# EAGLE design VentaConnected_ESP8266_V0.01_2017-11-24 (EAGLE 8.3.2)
VERSION: 0.01
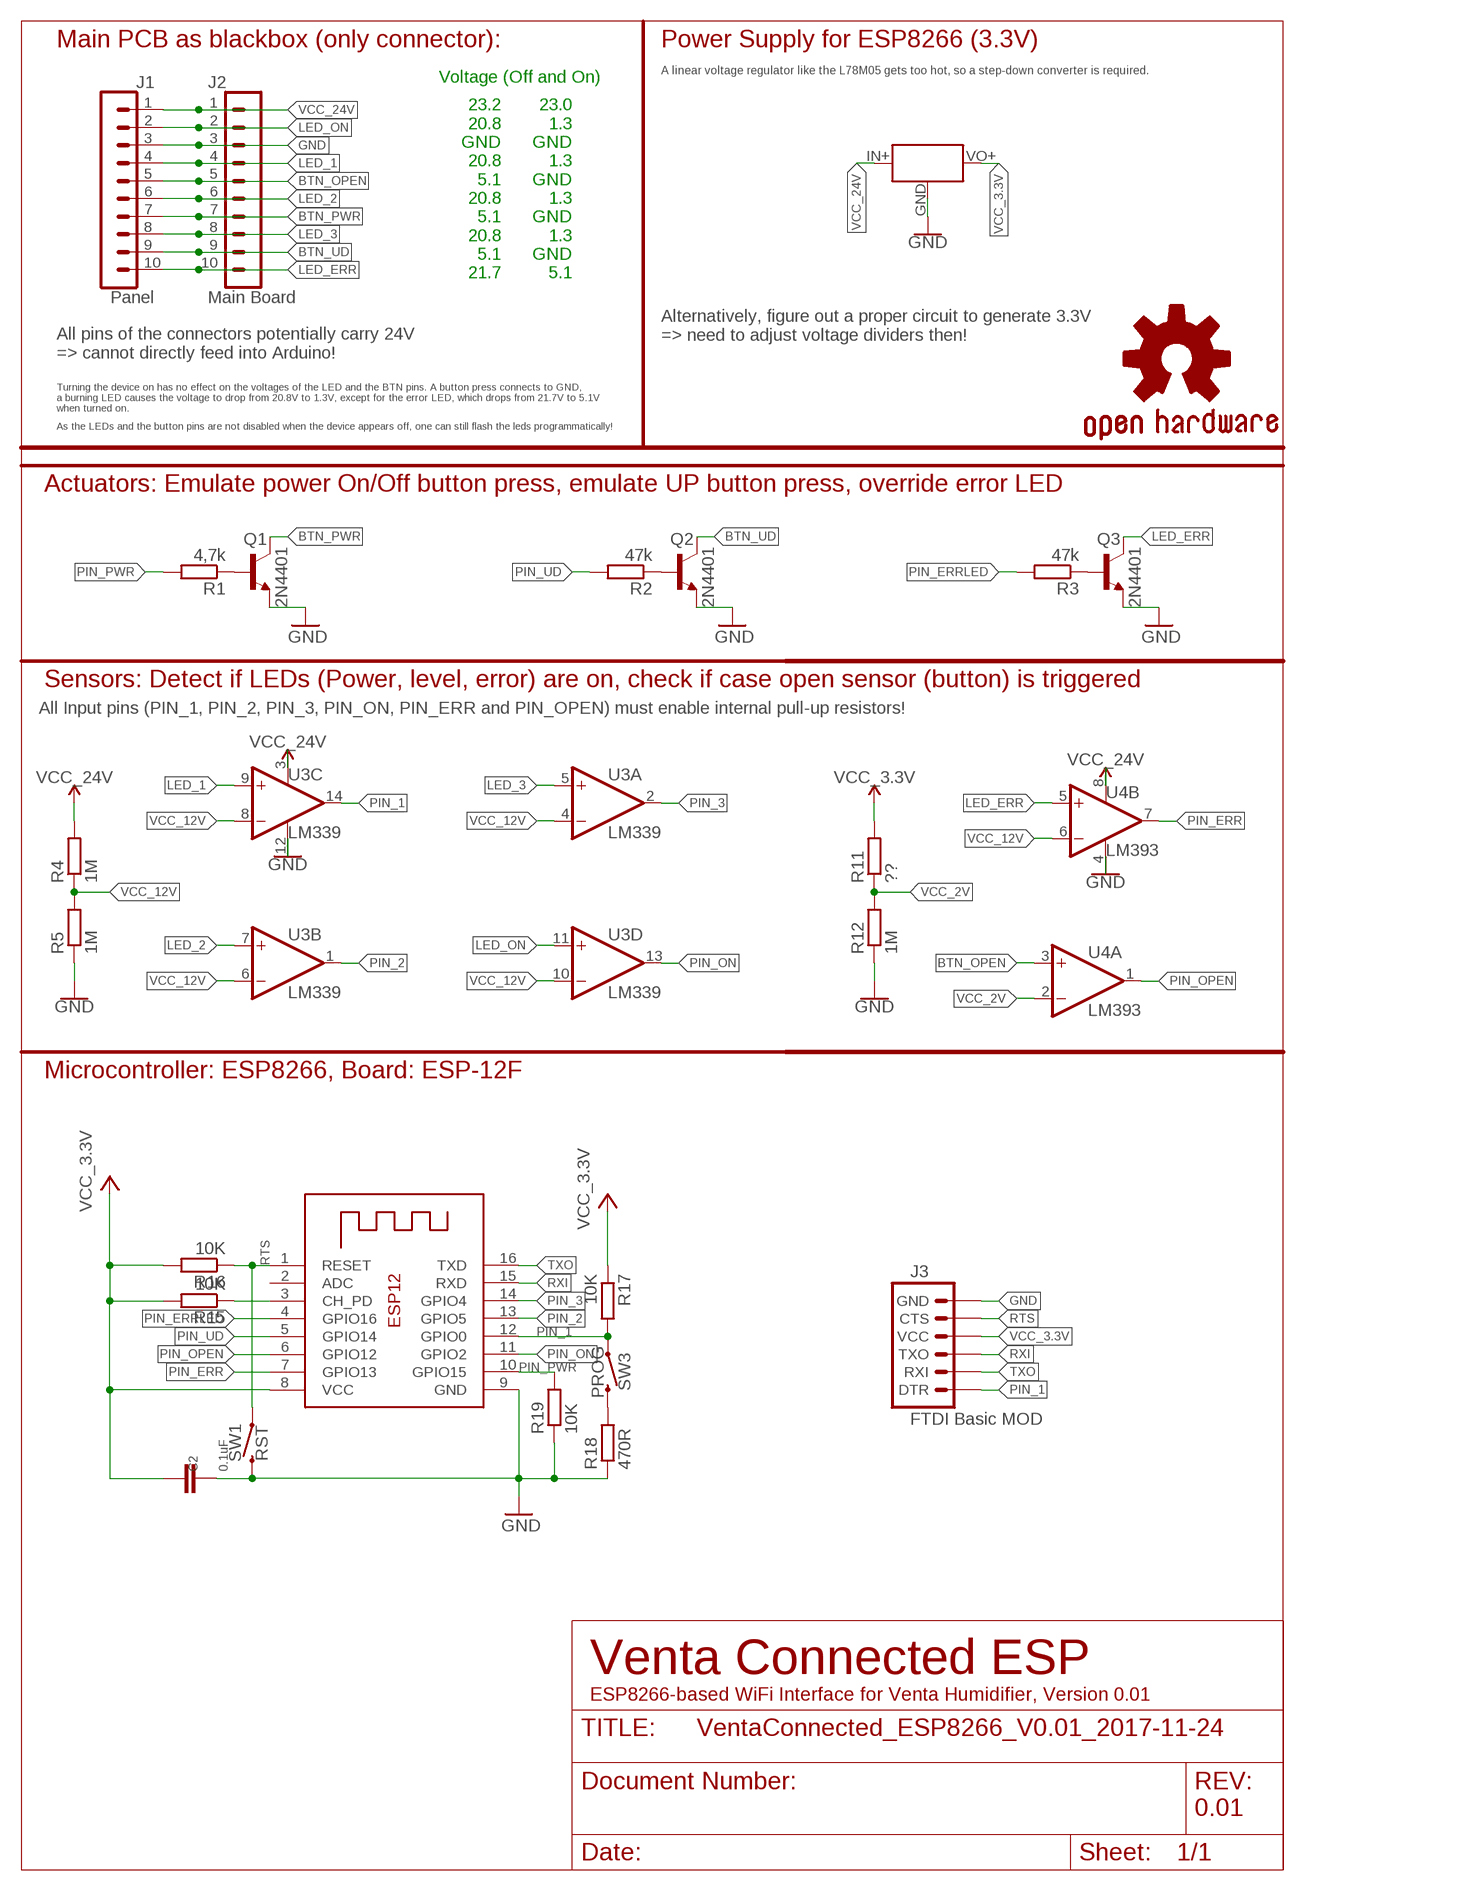
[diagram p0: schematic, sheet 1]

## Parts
C2  0.1uF  C-EUC0805  [C0805]
GOLD_ORB_SM1  OSHWLOGO_GOLD_ORB_SM  [OSHW2]
J1  Panel  CONN_05X2SHD  [2X5-SHROUDED]
J2  Main Board  CONN_05X2PTH  [2X5]
J3  FTDI Basic MOD  ARDUINO_SERIAL_PROGRAMPTH  [1X06]
Q1  2N4401  MMBT4401LT1-NPN-SOT23-BEC  [SOT23-BEC]
Q2  2N4401  MMBT4401LT1-NPN-SOT23-BEC  [SOT23-BEC]
Q3  2N4401  MMBT4401LT1-NPN-SOT23-BEC  [SOT23-BEC]
R1  4,7k  R-EU_R0805  [R0805]
R2  47k  R-EU_R0805  [R0805]
R3  47k  R-EU_R0805  [R0805]
R4  1M  R-EU_R0805  [R0805]
R5  1M  R-EU_R0805  [R0805]
R11  ??  R-EU_R0805  [R0805]
R12  1M  R-EU_R0805  [R0805]
R15  10K  R-EU_R0805  [R0805]
R16  10K  R-EU_R0805  [R0805]
R17  10K  R-EU_R0805  [R0805]
R18  470R  R-EU_R0805  [R0805]
R19  10K  R-EU_R0805  [R0805]
SW1  RST  MOMENTARY-SWITCH-SPST-SMD-6.0X3.5MM  [TACTILE_SWITCH_SMD_6.0X3.5MM]
SW3  PROG  MOMENTARY-SWITCH-SPST-SMD-6.0X3.5MM  [TACTILE_SWITCH_SMD_6.0X3.5MM]
U2  3.3V_BUCK_CONVERTER  MINI_BUCK_CONVERTER_UPSIDEDOWN  [MINI_BUCK_CONVERTER_UPDOWN]
U3  LM339  TLC339D  [SO14]
U4  LM393  LM393D  [SO08]
X2  ESP-12e  ESP-12  [ESP-12]

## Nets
BTN_OPEN: J1.5 J2.5 U4.3(A:+IN)
BTN_PWR: J1.7 J2.7 Q1.C
BTN_UD: J1.9 J2.9 Q2.C
CH_PD: R15.1 X2.3(CH_PD)
GND: C2.1 J1.3 J2.3 J3.6(GND) Q1.E Q2.E Q3.E R5.1 R12.1 R18.1 R19.1 SW1.2 U2.GND U3.12(P:V-) U4.4(P:V-) X2.9(GND)
LED_1: J1.4 J2.4 U3.9(C:+IN)
LED_2: J1.6 J2.6 U3.7(B:+IN)
LED_3: J1.8 J2.8 U3.5(A:+IN)
LED_ERR: J1.10 J2.10 Q3.C U4.5(B:+IN)
LED_ON: J1.2 J2.2 U3.11(D:+IN)
N$2: Q1.B R1.1
N$4: R18.2 SW3.2
N$5: Q3.B R3.1
N$6: Q2.B R2.1
PIN_1: J3.1(DTR) R17.2 SW3.1 U3.14(C:OUT) X2.12(GPIO0)
PIN_2: U3.1(B:OUT) X2.13(GPIO5)
PIN_3: U3.2(A:OUT) X2.14(GPIO4)
PIN_ERR: U4.7(B:OUT) X2.7(GPIO13)
PIN_ERRLED: R3.2 X2.4(GPIO16)
PIN_ON: U3.13(D:OUT) X2.11(GPIO2)
PIN_OPEN: U4.1(A:OUT) X2.6(GPIO12)
PIN_PWR: R1.2 R19.2 X2.10(GPIO15)
PIN_UD: R2.2 X2.5(GPIO14)
RTS: J3.5(CTS) R16.1 SW1.1 X2.1(RESET)
RXI: J3.3(TXO) X2.15(RXD)
TXO: J3.2(RXI) X2.16(TXD)
VCC_2V: R11.1 R12.2 U4.2(A:-IN)
VCC_3.3V: C2.2 J3.4(VCC) R11.2 R15.2 R16.2 R17.1 U2.VO+(VOUT) X2.8(VCC)
VCC_12V: R4.1 R5.2 U3.4(A:-IN) U3.6(B:-IN) U3.8(C:-IN) U3.10(D:-IN) U4.6(B:-IN)
VCC_24V: J1.1 J2.1 R4.2 U2.IN+(VIN) U3.3(P:V+) U4.8(P:V+)
Unconnected: X2.2(ADC)

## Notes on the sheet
- Main PCB as blackbox (only connector): | Power Supply for ESP8266 (3.3V)
- A linear voltage regulator like the L78M05 gets too hot, so a step-down converter is required.
- Voltage (Off and On)
- 23.2
  20.8
  GND
  20.8
  5.1
  20.8
  5.1
  20.8
  5.1
  21.7
- 23.0
  1.3
  GND
  1.3
  GND
  1.3
  GND
  1.3
  GND
  5.1
- Alternatively, figure out a proper circuit to generate 3.3V 
  => need to adjust voltage dividers then!
- All pins of the connectors potentially carry 24V 
  => cannot directly feed into Arduino!
- Turning the device on has no effect on the voltages of the LED and the BTN pins. A button press connects to GND, 
  a burning LED causes the voltage to drop from 20.8V to 1.3V, except for the error LED, which drops from 21.7V to 5.1V 
  when turned on.
- As the LEDs and the button pins are not disabled when the device appears off, one can still flash the leds programmatically!
- Actuators: Emulate power On/Off button press, emulate UP button press, override error LED
- Sensors: Detect if LEDs (Power, level, error) are on, check if case open sensor (button) is triggered
- All Input pins (PIN_1, PIN_2, PIN_3, PIN_ON, PIN_ERR and PIN_OPEN) must enable internal pull-up resistors!
- Microcontroller: ESP8266, Board: ESP-12F
- Venta Connected ESP
- ESP8266-based WiFi Interface for Venta Humidifier, Version 0.01

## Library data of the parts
C2 = resistor:C-EU: CAPACITOR, European symbol
GOLD_ORB_SM1 = bfl:OSHWLOGO: These are Open-Source Hardware logos.
J1 = opentools-connectors:CONN_05X2: Multi connection point. Often used as Generic Header-pin footprint for 0.1 inch spaced/style header connections For AVR SPI programming port, see special device with nice symbol: "AVR_SPI_PROG_5x2.dev" You can populate with any combo of single row headers, but if you'd like an exact match, check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; PROD_ID: CONN-08671; SF_ID: PRT-08506
J2 = opentools-connectors:CONN_05X2: Multi connection point. Often used as Generic Header-pin footprint for 0.1 inch spaced/style header connections For AVR SPI programming port, see special device with nice symbol: "AVR_SPI_PROG_5x2.dev" You can populate with any combo of single row headers, but if you'd like an exact match, check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; PROD_ID: CONN-08499; SF_ID: PRT-0778
J3 = SparkFun:ARDUINO_SERIAL_PROGRAM
Q1-Q3 = transistor-neu-to92:*-NPN-: NPN Transistror
R1-R5 R11 R12 = resistor:R-EU_: RESISTOR, European symbol
R15-R19 = rcl:R-EU_: RESISTOR, European symbol
SW1 SW3 = SparkFun-Switches:MOMENTARY-SWITCH-SPST: Momentary Switch (Pushbutton) - SPST; PROD_ID: SWCH-00815; SF_SKU: COM-08229
U2 = opentools-sensors:MINI_BUCK_CONVERTER: 4.5-40V Step Down Buck Converter
U3 = linear:TLC339: COMPARATOR
U4 = linear:LM393: COMPARATOR
X2 = adafruit:ESP-12

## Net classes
0 default: width 0.203 mm
1 vcc: width 0.254 mm

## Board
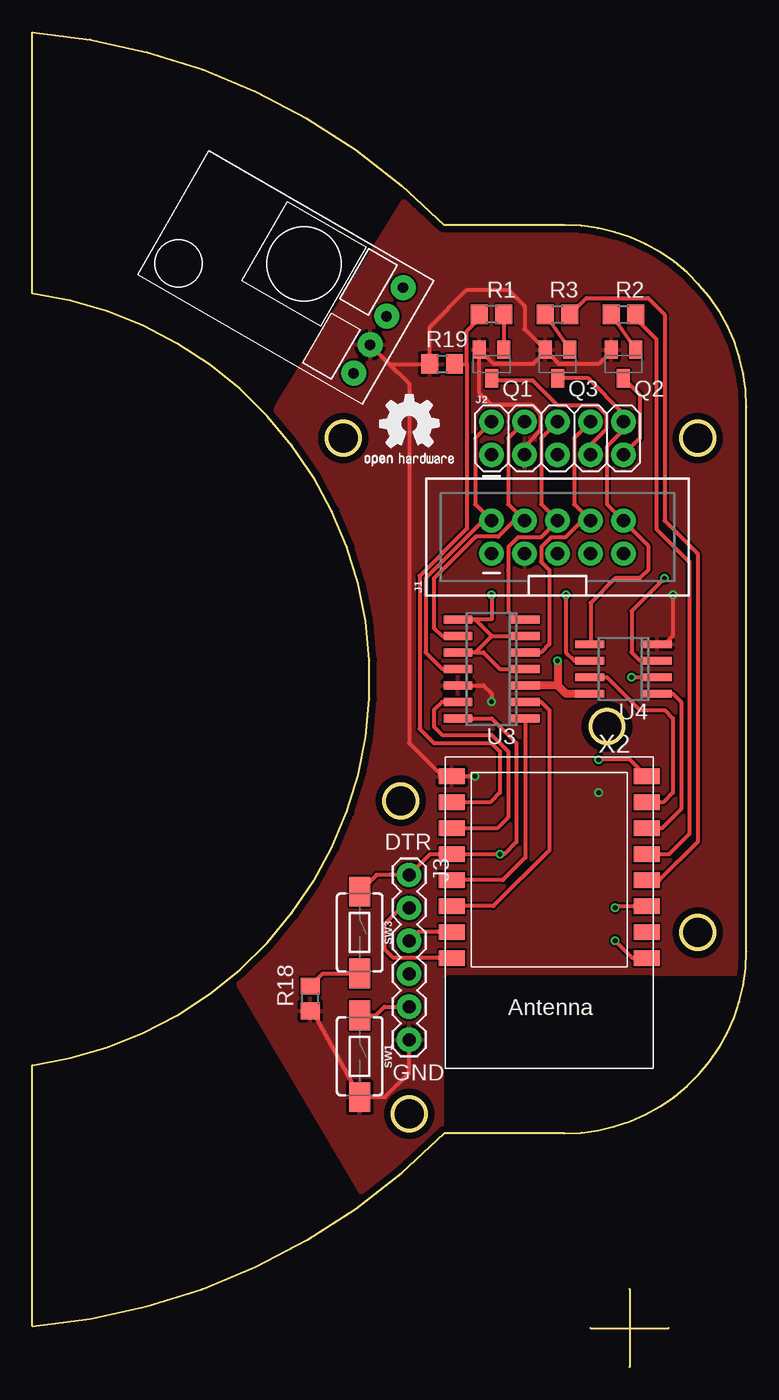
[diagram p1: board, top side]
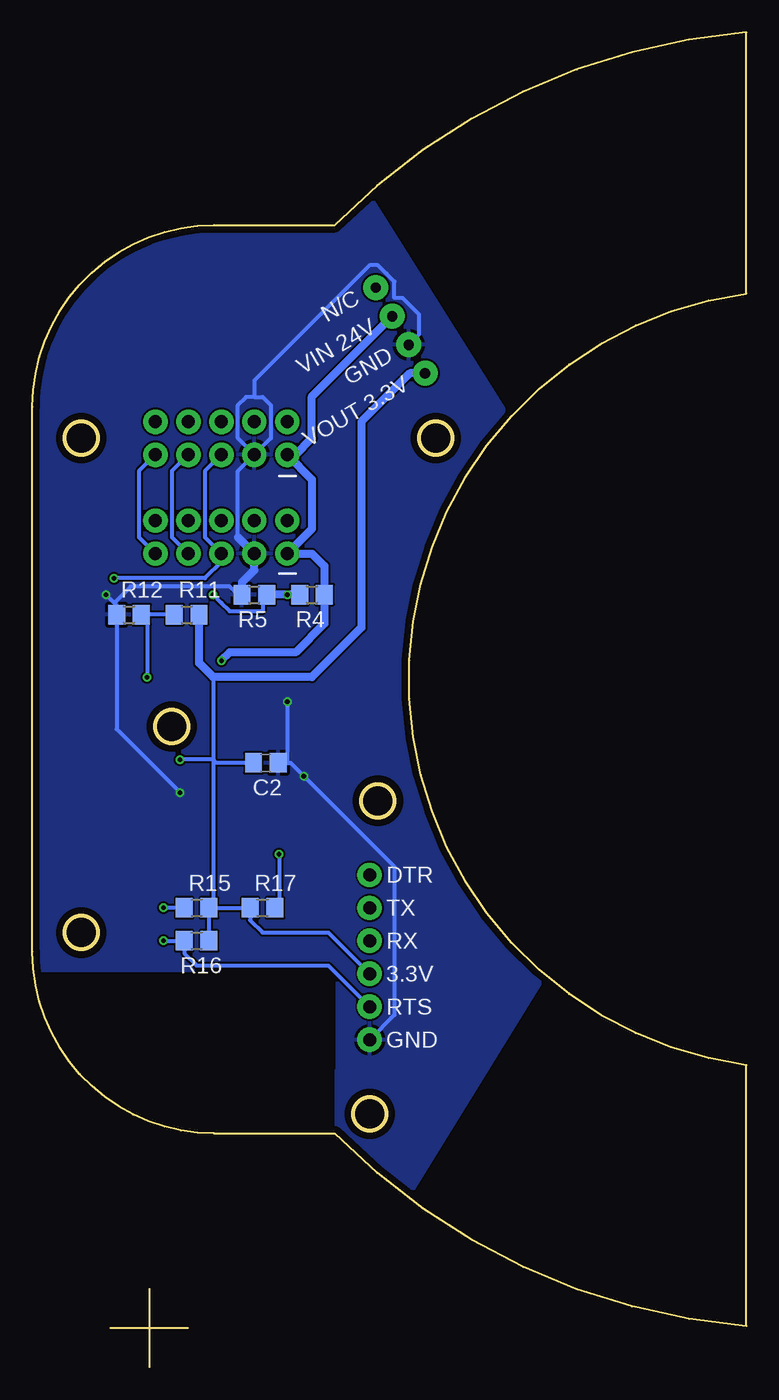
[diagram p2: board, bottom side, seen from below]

Size 55 x 102.85 mm. Coordinates in mm from the lower left corner, seen from the top.
Outline: 46,6 46,0
Outline: 43,3 49,3
Outline: 41,18 arc90 55,32 55,74 arc90 41,88 31.71,88 arc41 0,102.85 0,82.73 arc-165 0,23.27 0,3.16 arc41 31.71,18 41,18
Outline: circle at 29.02,19.51 radius 1.27
Outline: circle at 51.24,33.48 radius 1.27
Outline: circle at 28.38,43.64 radius 1.27
Outline: circle at 51.24,71.58 radius 1.27
Outline: circle at 23.94,71.58 radius 1.27
Outline: circle at 44.26,49.35 radius 1.27
Copper layers (1*16): Top 0.035mm / dielectric 1.6mm / Bottom 0.035mm
Design rules "Elecrow_2-layer_PCB_eagle_rule": minimum track width 6mil, minimum drill 12mil, track to track 6mil, track to pad 6mil, pad to pad 6mil, via to via 8mil, smd to smd 0mil, copper to edge 20mil, drill to drill 10mil, minimum pad ring 6mil, minimum via ring 6mil, stop-mask expansion 0mil, vias tented up to drill 100mil, thermal gap 10mil

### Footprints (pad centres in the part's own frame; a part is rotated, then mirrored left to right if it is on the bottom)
C0805 = smd 1.3 x 1.5: 1 -0.95,0; 2 0.95,0
2X5-SHROUDED = drill 1.016 pad 1.88: 1 -1.27,5.08; 2 1.27,5.08; 3 -1.27,2.54; 4 1.27,2.54; 5 -1.27,0; 6 1.27,0; 7 -1.27,-2.54; 8 1.27,-2.54; 9 -1.27,-5.08; 10 1.27,-5.08
2X5 = drill 1.016 pad 1.88: 1 0,0; 2 0,2.54; 3 2.54,0; 4 2.54,2.54; 5 5.08,0; 6 5.08,2.54; 7 7.62,0; 8 7.62,2.54; 9 10.16,0; 10 10.16,2.54
1X06 = drill 1.016 pad 1.88: 1 0,0; 2 2.54,0; 3 5.08,0; 4 7.62,0; 5 10.16,0; 6 12.7,0
SOT23-BEC = smd 1 x 1.4: B -0.95,-1.1; C 0,1.1; E 0.95,-1.1
R0805 = smd 1.3 x 1.5: 1 -0.95,0; 2 0.95,0
TACTILE_SWITCH_SMD_6.0X3.5MM = smd 2.3 x 1.6: 1 -3.15,0; 2 3.15,0
MINI_BUCK_CONVERTER_UPDOWN = drill 0.8 pad 1.93: EN -1.27,1.27; GND -6.35,1.27; IN+ -3.81,1.27; VO+ -8.89,1.27
SO14 = smd 0.6 x 2.2: 1 -3.81,-2.6; 2 -2.54,-2.6; 3 -1.27,-2.6; 4 0,-2.6; 5 1.27,-2.6; 6 2.54,-2.6; 7 3.81,-2.6; 8 3.81,2.6; 9 2.54,2.6; 10 1.27,2.6; 11 0,2.6; 12 -1.27,2.6; 13 -2.54,2.6; 14 -3.81,2.6
SO08 = smd 0.6 x 2.2: 1 -1.905,-2.6; 2 -0.635,-2.6; 3 0.635,-2.6; 4 1.905,-2.6; 5 1.905,2.6; 6 0.635,2.6; 7 -0.635,2.6; 8 -1.905,2.6
ESP-12 = smd 2 x 1.2: 1 -7.5,4.5; 2 -7.5,2.5; 3 -7.5,0.5; 4 -7.5,-1.5; 5 -7.5,-3.5; 6 -7.5,-5.5; 7 -7.5,-7.5; 8 -7.5,-9.5; 9 7.5,-9.5; 10 7.5,-7.5; 11 7.5,-5.5; 12 7.5,-3.5; 13 7.5,-1.5; 14 7.5,0.5; 15 7.5,2.5; 16 7.5,4.5

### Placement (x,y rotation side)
C2  37.02,46.56 180 bottom
GOLD_ORB_SM1  25.21,68.41 0 top
J1  40.45,63.96 90 top
J2  35.37,70.31 0 top
J3  29.02,37.92 270 top
Q1  35.37,77.3 180 top
Q2  45.53,77.3 180 top
Q3  40.45,77.3 180 top
R1  35.37,81.11 180 top
R2  45.53,81.11 0 top
R3  40.45,81.11 0 top
R4  33.47,59.52 0 bottom
R5  37.91,59.52 0 bottom
R11  43.12,57.99 0 bottom
R12  47.56,57.99 0 bottom
R15  42.35,35.38 0 bottom
R16  42.35,32.84 0 bottom
R17  37.27,35.38 0 bottom
R18  21.4,28.4 90 top
R19  31.56,77.3 0 top
SW1  25.21,23.95 270 top
SW3  25.21,33.48 270 top
U2  30.29,83.64 60 top
U3  35.37,53.8 90 top
U4  45.53,53.8 90 top
X2  39.81,36.02 180 top

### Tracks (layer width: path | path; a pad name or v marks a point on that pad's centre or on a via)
BTN_OPEN  (via drill 0.35)
  Top 0.305: v48.7,60.78 46.16,58.24 46.16,55.07 46.8,54.44 U4.3
  Bottom 0.305: J2.5 41.72,69.04 41.72,63.96 J1.5 40.45,62.05 41.72,60.78 v48.7,60.78
BTN_PWR
  Top 0.305: Q1.C 35.54,76.03 38.55,76.03 40.48,74.09 43.51,74.09 44.23,73.37 44.23,72.33 42.99,71.09 J2.7
  Bottom 0.305: J2.7 44.26,69.04 44.26,63.96 J1.7
BTN_UD
  Top 0.305: 45.53,76.03 Q2.C 46.8,74.92 46.8,71.58 J2.9
  Bottom 0.305: J2.9 46.8,69.04 46.8,63.96 J1.9
CH_PD  (via drill 0.35)
  Top 0.305: v44.9,35.38 45.03,35.52 X2.3
  Bottom 0.305: R15.1 v44.9,35.38
GND  (via drill 0.35)
  Top 0.305: 32.34,45.55 v34.1,45.55 | 32.34,45.55 X2.9 | R18.1 21.75,27.11 SW1.2 27.14,20.8 29.02,22.68 J3.6 | J2.3 37.91,70.94 38.72,71.76 38.72,71.77 39.17,72.22 39.17,73.49 38.55,74.12 35.37,74.12 34.42,75.07 Q1.E 35.52,77.3 38.55,77.3 39.5,78.25 Q3.E 39.57,78.32 | v49.34,59.52 49.34,56.34 48.7,55.7 U4.4 | U3.12 34.73,52.53 35.37,51.9 v35.37,51.26 | Q2.E 44.58,78.25 43.62,77.3 40.6,77.3 39.57,78.32 | U2.GND 27.31,77.49 | 27.31,77.49 27.5,77.3 R19.1 30.61,80.16 33.47,83.01 36.64,83.01 37.91,81.74 37.91,79.98 39.57,78.32 | 27.31,77.49 29.02,75.78 29.02,48.09 31.56,45.55 32.34,45.55
  Bottom 0.305: J2.3 39.18,69.04 39.18,63.96 | 35.37,46.56 C2.1 | 35.37,46.56 35.12,46.56 v34.1,45.55 27.11,38.56 27.11,27.13 J3.6 | J2.3 39.18,71.58 39.18,74.12 38.55,74.75 37.91,74.75 | J2.3 36.64,71.58 36.64,74.12 37.27,74.75 37.91,74.75 | v35.37,51.26 35.37,46.56 | 48.7,58.88 48.51,58.69 R12.1 48.51,49.16 v43.62,44.27 | 48.7,58.88 v49.34,59.52 | R5.1 39.18,59.52 39.81,60.15 47.44,60.15 48.7,58.88 | U2.GND 25.21,79.59 25.21,81.11 26.48,82.38 27.11,82.38 27.11,83.64 27.69,84.22 27.72,84.27 27.75,84.28 28.38,84.92 29.02,84.92 37.91,76.03 37.91,74.75
  Bottom 0.61: R5.1 38.86,60.47 37.91,61.42 J1.3 39.18,63.96
  pour Top (isolate 0.152): 29.02,90.63 18.86,74.12 18.23,72.85 22.04,67.14 24.57,62.05 25.84,53.8 25.21,46.18 20.77,36.02 15.68,29.67 25.84,12.53 31.56,16.97 31.56,30.3 55.05,30.3 55.69,74.12 51.88,84.28 42.99,88.09 31.56,88.09
  pour Bottom (isolate 0.152): 29.02,90.25 18.23,73.1 20.13,69.93 23.94,62.31 25.84,55.32 25.21,45.8 19.5,34.37 15.68,29.92 25.84,13.41 29.02,15.32 31.56,17.86 31.56,30.56 55.05,30.56 55.69,73.74 51.88,83.9 42.99,87.71 31.56,87.71
LED_1
  Top 0.305: J2.4 36.64,71.58 36.64,66.5 J1.4 37.13,65.23 35.89,63.98 34.14,63.98 34.11,63.95 | 34.11,63.95 34.11,63.96 | 34.11,63.95 30.93,60.78 30.93,56.97 31.56,56.34 U3.9
LED_2
  Top 0.305: J2.6 39.18,71.58 39.18,66.5 J1.6 39.16,63.94 37.39,63.94 36.66,63.21 36.66,61.45 | 36.64,61.42 36.66,61.45 | 36.66,61.45 36.66,58.22 37.27,57.61 U3.7
LED_3
  Top 0.305: J2.8 41.72,71.58 41.72,66.5 J1.8 42.35,65.23 41.06,63.94 39.93,63.94 39.2,63.21 39.2,62.08 39.18,62.05 39.81,61.42 39.81,55.7 39.18,55.07 U3.5
LED_ERR
  Top 0.305: Q3.C 42.82,76.19 45.53,73.48 J2.10 45.53,72.22 44.26,70.94 44.26,66.5 J1.10 47.44,63.33 47.44,61.42 46.8,60.78 44.9,60.78 42.99,58.88 42.99,55.77 U4.5
LED_ON
  Top 0.305: J2.2 34.1,71.58 34.1,66.5 J1.2 34.73,65.23 30.29,60.78 30.29,55.07 31.56,53.8 U3.11
N$2
  Top 0.305: R1.1 Q1.B
N$4
  Top 0.305: R18.2 22.38,30.33 SW3.2
N$5
  Top 0.305: R3.1 Q3.B
N$6
  Top 0.305: R2.1 Q2.B
PIN_1  (via drill 0.35)
  Top 0.305: U3.14 35.37,49.99 37.27,48.09 37.27,40.47 36.33,39.52 v36.01,39.52 X2.12 30.62,39.52 J3.1 26.5,37.92 SW3.1
  Bottom 0.305: v36.01,39.52 36.01,35.7 R17.2
PIN_2
  Top 0.305: U3.1 37.97,39.26 36.23,37.52 X2.13
PIN_3
  Top 0.305: U3.2 39.18,51.26 39.81,50.62 39.81,39.83 35.51,35.52 X2.14
PIN_ERR
  Top 0.305: U4.7 44.26,53.16 46.8,50.62 48.7,50.62 49.34,49.99 49.34,44.27 48.59,43.52 X2.7
PIN_ERRLED
  Top 0.305: R3.2 42.67,82.38 47.44,82.38 48.7,81.11 48.7,65.23 51.24,62.69 51.24,40.47 48.3,37.52 X2.4
PIN_ON
  Top 0.305: U3.13 31.56,51.26 30.92,50.62 30.92,49.35 31.56,48.72 35.37,48.72 36.64,47.45 36.64,42.37 35.79,41.52 X2.11
PIN_OPEN
  Top 0.305: U4.1 49.34,51.9 49.98,51.26 49.98,43.01 48.49,41.52 X2.6
PIN_PWR
  Top 0.305: R1.2 34.42,80.79 33.47,79.83 33.47,77.3 | 33.47,77.3 33.47,64.61 29.83,60.97 29.83,49.18 30.92,48.09 35.36,48.09 36.01,47.44 36.01,44.27 35.25,43.52 X2.10 | R19.2 33.47,77.3
PIN_UD
  Top 0.305: R2.2 46.48,80.79 48.07,79.2 48.07,64.59 50.61,62.05 50.61,41.1 49.03,39.52 X2.5
RTS  (via drill 0.35)
  Top 0.305: X2.1 46.22,31.52 v44.9,32.84 | SW1.1 26.45,27.11 27.11,27.77 J3.5
  Bottom 0.305: v44.9,32.84 R16.1 43.3,31.89 42.35,30.94 32.2,30.94 J3.5
RXI
  Top 0.305: X2.15 29.7,33.52 J3.3
TXO
  Top 0.305: J3.2 28.38,35.38 27.11,34.11 27.11,32.21 27.75,31.57 32.26,31.57 X2.16
VCC_2V  (via drill 0.35)
  Top 0.305: v46.16,53.16 U4.2
  Bottom 0.305: R11.1 R12.2 46.16,57.54 v46.16,53.16
VCC_3.3V  (via drill 0.35)
  Top 0.305: v43.62,46.81 46.02,46.81 X2.8
  Bottom 0.305: 41.09,35.38 R17.1 38.23,34.43 37.27,33.48 32.2,33.48 J3.4 | 41.09,35.38 R15.2 R16.2 | 41.09,53.16 41.09,46.81 | 41.09,46.81 41.09,35.38 | C2.2 40.83,46.56 41.09,46.81 | 41.09,46.81 v43.62,46.81
  Bottom 0.61: U2.VO+ 25.92,76.58 29.66,72.85 29.66,56.98 33.47,53.16 41.09,53.16 42.17,54.25 R11.2
VCC_12V  (via drill 0.35)
  Top 0.305: 34.1,57.61 35.37,56.34 | 35.37,56.34 U3.6 | 35.37,56.34 34.1,55.07 | 34.1,55.07 U3.10 | 34.1,55.07 34.73,55.07 36.01,53.8 U3.4 | v35.37,59.52 35.37,57.61 34.1,57.61 | 34.1,57.61 32.83,57.61 | v41.09,59.52 41.09,55.07 41.72,54.44 U4.6 | U3.8 34.1,57.61
  Bottom 0.305: R5.2 37.27,59.2 37.27,58.24 39.81,58.24 40.45,58.88 v41.09,59.52
  Bottom 0.61: R4.1 v35.37,59.52 R5.2
VCC_24V  (via drill 0.35)
  Top 0.61: v40.45,54.44 40.45,52.53 | 40.45,52.53 U3.3 | 40.45,52.53 41.09,51.9 U4.8
  Bottom 0.61: U2.IN+ 33.47,74.8 33.47,71.58 34.73,70.31 J2.1 33.47,68.41 33.47,64.59 J1.1 33.47,62.69 32.52,61.74 R4.2 32.52,57.29 34.73,55.07 39.81,55.07 v40.45,54.44

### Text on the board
tOrigins: PROG | RESET
bOrigins: VentaConnected for ESP8266 / R. Kainhofer / Version 0.01, 26.11.2017
tNames: DTR | GND
bNames: N/C / VIN 24V / GND / VOUT 3.3V | DTR / TX / RX / 3.3V / RTS / GND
